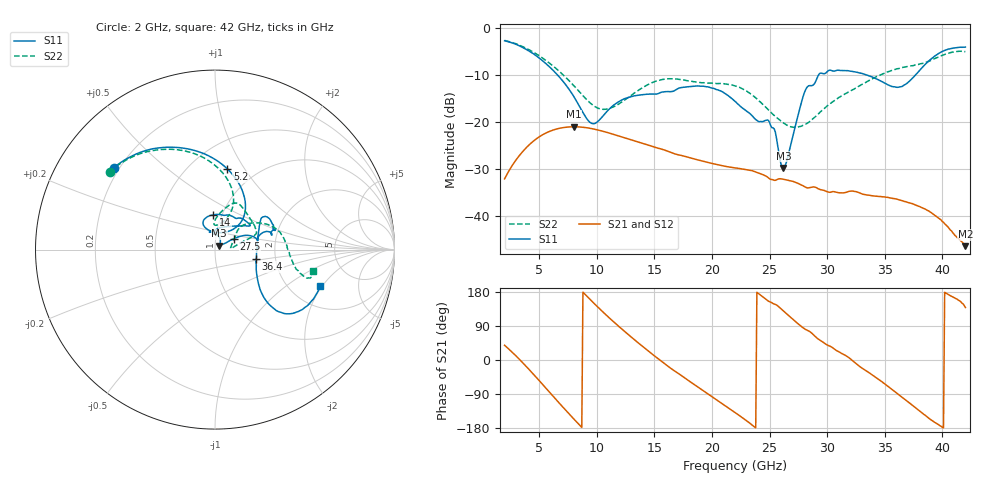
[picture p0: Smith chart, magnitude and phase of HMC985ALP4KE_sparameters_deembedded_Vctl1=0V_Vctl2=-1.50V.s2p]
!s2p File: Measurements: S11, S21, S12, S22
# GHz S dB R 50.0
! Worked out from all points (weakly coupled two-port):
!   401 points, 2 GHz to 42 GHz, reference 50 ohm
!   highest |S21| = -21.05 dB at 8 GHz (marker M1); lowest = -46.4 dB at 42 GHz (marker M2)
!   lowest |S11| = -29.8 dB at 26.2 GHz (marker M3), VSWR 1.07, Z = 52.4 + j2.31 ohm
!   |S11| at or under -10 dB: 6.571 GHz to 29.27 GHz (22.7 GHz wide, 127 % of centre); 33.35 GHz to 37.69 GHz (4.341 GHz wide, 12.2 % of centre)
!   |S22| runs from -21.2 to -2.7 dB; largest |S21 - S12| = 0.00014
!   S11 on the Smith chart (normalised r, x): 2 GHz: 0.18, +0.34; 5.2 GHz: 0.74, +0.84; 14 GHz: 0.91, +0.37; 27.5 GHz: 1.22, +0.15; 36.4 GHz: 1.58, -0.18; 42 GHz: 2.90, -1.91
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2  -2.79 140.9  -32.12 38.9  -32.12 38.8  -2.73 143.5
3.5  -4.14 113.3  -26.52 -5.0  -26.52 -5.0  -3.96 118.3
5.2  -6.85 81.2  -22.90 -61.1  -22.90 -61.1  -6.31 92.1
8  -14.61 46.2  -21.05 -155.4  -21.06 -155.4  -12.31 67.1
8.7  -17.61 52.0  -21.14 -177.8  -21.14 -177.8  -14.20 68.7
9.7  -20.41 84.4  -21.51 151.3  -21.51 151.3  -16.55 78.0
10.8  -18.03 112.2  -22.19 119.1  -22.20 119.1  -17.33 89.9
14  -14.24 92.5  -24.57 35.3  -24.58 35.3  -12.72 77.3
15.4  -13.94 73.0  -25.65 1.9  -25.66 1.9  -11.18 68.7
19.4  -12.52 34.4  -28.49 -84.2  -28.49 -84.2  -11.74 37.8
22  -15.64 52.3  -29.79 -138.3  -29.80 -138.3  -12.38 20.4
25  -20.15 98.1  -32.10 153.8  -32.10 153.8  -17.72 12.6
26.2  -29.78 42.7  -32.20 129.1  -32.20 129.1  -20.24 5.5
27.5  -18.38 29.9  -33.12 94.9  -33.13 94.8  -21.08 6.9
28.1  -13.34 20.8  -33.86 81.1  -33.87 81.1  -20.56 13.7
28.7  -12.30 12.9  -33.85 69.8  -33.85 69.8  -19.50 21.5
31  -9.07 23.3  -35.07 21.8  -35.06 21.9  -14.86 41.6
33.3  -9.95 34.3  -35.47 -26.7  -35.48 -26.8  -11.71 34.7
35.4  -12.27 12.3  -36.13 -72.4  -36.11 -72.4  -9.31 22.3
36.4  -12.57 -12.9  -36.67 -96.0  -36.70 -96.0  -8.53 15.1
39.5  -5.81 -43.3  -40.17 -167.5  -40.15 -167.9  -6.40 -14.2
42  -4.14 -19.0  -46.41 138.4  -46.38 139.6  -5.09 -12.4
